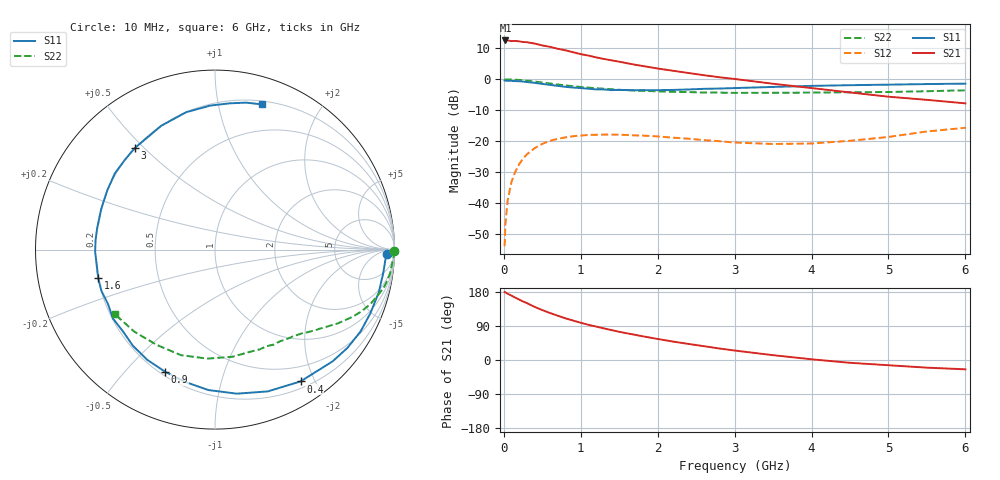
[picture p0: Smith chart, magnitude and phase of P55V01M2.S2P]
! SIEMENS Small Signal Semiconductors
! BFP183
! Si NPN RF Bipolar Junction Transistor in SOT143
! VCE = 5 V  IC = 1.2 mA
! Common Emitter S-Parameters:  March  1996
# GHz  S  MA  R  50
!  f  S11  S21  S12  S22
! GHz  MAG  ANG  MAG  ANG  MAG  ANG  MAG  ANG
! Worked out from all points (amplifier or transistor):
!   36 points, 10 MHz to 6 GHz, reference 50 ohm
!   highest |S21| = 12.6 dB at 20 MHz (marker M1)
!   |S21| within 3 dB of that: start of sweep to 763.9 MHz
!   unconditionally stable (mu >= 1): 2.435 GHz to end of sweep
!   at 250 MHz: K = 0.09, MSG = 18.9 dB, |S12| = -25.7 dB
!   at 1.4 GHz: K = 0.56, MSG = 12.0 dB, |S12| = -17.9 dB
!   at 6 GHz: K = 1.04, MAG = 2.8 dB, |S12| = -15.7 dB
!   S11 on the Smith chart (normalised r, x): 10 MHz: 35, -19; 400 MHz: 0.29, -1.81; 900 MHz: 0.22, -0.65; 1.6 GHz: 0.20, -0.11; 3 GHz: 0.20, +0.47; 6 GHz: 0.23, +1.35
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0.01  0.9572 -1.4  4.201 179.3  0.002 84.5  0.9995 -0.5
0.02  0.9514 -3.1  4.247 178.5  0.0045 84.1  0.9972 -1.1
0.05  0.9468 -7.6  4.244 174.8  0.0111 88.3  0.9955 -2.5
0.1  0.9432 -14.6  4.149 169.8  0.022 80.9  0.9885 -5.2
0.15  0.9355 -22.4  4.177 164.5  0.0322 75.9  0.984 -7.8
0.25  0.9188 -36.6  4.007 154.4  0.0521 68.7  0.9637 -12.7
0.3  0.904 -43.5  3.976 150.1  0.0612 64.4  0.9484 -14.8
0.4  0.8756 -57.0  3.785 140.2  0.0769 56.8  0.9191 -19.1
0.5  0.843 -69.6  3.528 131.6  0.0902 49.7  0.8873 -22.7
0.6  0.8118 -81.4  3.348 124.0  0.1011 43.6  0.8558 -25.8
0.8  0.7556 -102.8  2.945 110.0  0.1149 33.0  0.7972 -31.1
0.9  0.7349 -112.2  2.739 104.1  0.1199 28.7  0.7715 -33.2
1.1  0.7045 -130.5  2.415 92.8  0.1258 21.3  0.7323 -36.9
1.3  0.6861 -146.0  2.132 83.4  0.1276 14.9  0.703 -40.3
1.6  0.6695 -166.5  1.822 70.4  0.1258 7.7  0.6676 -44.8
1.9  0.6676 175.4  1.568 59.1  0.1211 3.0  0.6443 -49.7
2.2  0.673 160.3  1.374 48.6  0.1137 -0.1  0.6262 -54.7
3  0.7209 128.4  1.012 25.0  0.0949 0.2  0.6027 -70.1
3.5  0.752 113.5  0.847 12.7  0.0899 6.7  0.6047 -80.9
4.5  0.8027 91.9  0.613 -7.4  0.1012 21.5  0.618 -107.9
5.5  0.8371 78.0  0.465 -20.2  0.1433 26.6  0.6413 -134.5
6  0.8502 72.1  0.408 -24.6  0.1644 23.8  0.6636 -147.1
